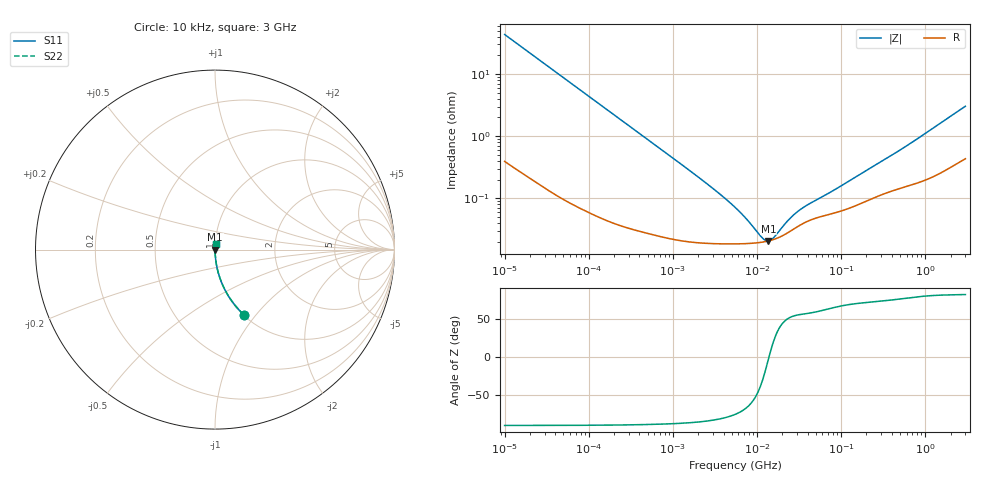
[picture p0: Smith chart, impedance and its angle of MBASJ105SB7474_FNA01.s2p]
! MBASJ105SB7474_FNA01  S-PARAMETER MODEL  ( Standard Model )
! Model Generated by TAIYO YUDEN Corporation (http://www.ty-top.com)
! Version 2.0
! TAIYO YUDEN Control No. 230906
! Copyright(c) 2013 TAIYO YUDEN CO.,LTD. All Rights Reserved.
! Product Description (link to TY-COMPAS)
! https://ds.yuden.co.jp/TYCOMPAS/or/detail?pn=MBASJ105SB7474KFNA01&u=M
! Products Name : Multilayer Ceramic Capacitors
! Characteristics :
!  Capacitance : 0.47 [uF] , Rated Voltage : 6.3 [V] , TCC : X7R
!  Case Size : 1.0 x 0.5 / 0.039 x 0.02 [mm/inch] , Thickness : 0.5 / 0.02 [mm/inch]
!  (Conditions: Temperature = 25 [degC] , DC Bias Voltage = 0 [V])
! External Node Assignments :
!  1  o---| |---o  2
! GND o---------o GND
! Frequency Range : 10kHz  -  3GHz  [ 401 STEP ]
# MHZ S RI R 50
! Freq[MHz].  S11 Real  S11 Imag  S21 Real  S21 Imag  S12 Real  S12 Imag  S22 Real  S22 Imag
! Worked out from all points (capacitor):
!   401 points, 10 kHz to 3 GHz, reference 50 ohm
!   read as one part in series: C = 367 nF near 10.65 kHz
!   lowest |Z| = 20.6 mohm at 13.67 MHz (marker M1)
!   series resonance near 13.88 MHz, so ESL is about 360 pH
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0.01  0.1602 -0.3623  0.8398 0.3623  0.8398 0.3623  0.1602 -0.3623
0.014599  0.0833 -0.2718  0.9167 0.2718  0.9167 0.2718  0.0833 -0.2718
0.021995  0.0393 -0.1896  0.9607 0.1896  0.9607 0.1896  0.0393 -0.1896
0.040039  0.0128 -0.1075  0.9872 0.1075  0.9872 0.1075  0.0128 -0.1075
0.082683  0.00346 -0.0528  0.9965 0.0528  0.9965 0.0528  0.00346 -0.0528
0.199902  0.000877 -0.022  0.9991 0.022  0.9991 0.022  0.000877 -0.022
0.683653  0.000287 -0.00649  0.9997 0.00649  0.9997 0.00649  0.000287 -0.00649
2.652321  0.00019 -0.00163  0.9998 0.00163  0.9998 0.00163  0.00019 -0.00163
5.477226  0.000185 -0.000693  0.9998 0.000693  0.9998 0.000693  0.000185 -0.000693
7.507384  0.000187 -0.000424  0.9998 0.000424  0.9998 0.000424  0.000187 -0.000424
11.31085  0.000196 -0.000134  0.9998 0.000134  0.9998 0.000134  0.000196 -0.000134
12.43293  0.0002 -7.19e-05  0.9998 7.19e-05  0.9998 7.19e-05  0.0002 -7.19e-05
13.66633  0.000206 -1.02e-05  0.9998 1.02e-05  0.9998 1.02e-05  0.000206 -1.02e-05
14.55585  0.00021 3.08e-05  0.9998 -3.08e-05  0.9998 -3.08e-05  0.00021 3.08e-05
15.99985  0.000219 9.23e-05  0.9998 -9.23e-05  0.9998 -9.23e-05  0.000219 9.23e-05
22.63272  0.000273 0.000318  0.9997 -0.000318  0.9997 -0.000318  0.000273 0.000318
28.22191  0.000329 0.000456  0.9997 -0.000456  0.9997 -0.000456  0.000329 0.000456
35.19136  0.000392 0.000586  0.9996 -0.000586  0.9996 -0.000586  0.000392 0.000586
45.28751  0.000458 0.000734  0.9995 -0.000734  0.9995 -0.000734  0.000458 0.000734
87.80663  0.000593 0.0013  0.9994 -0.0013  0.9994 -0.0013  0.000593 0.0013
374.4521  0.00129 0.0045  0.9987 -0.0045  0.9987 -0.0045  0.00129 0.0045
3000  0.0052 0.0297  0.9948 -0.0297  0.9948 -0.0297  0.0052 0.0297
